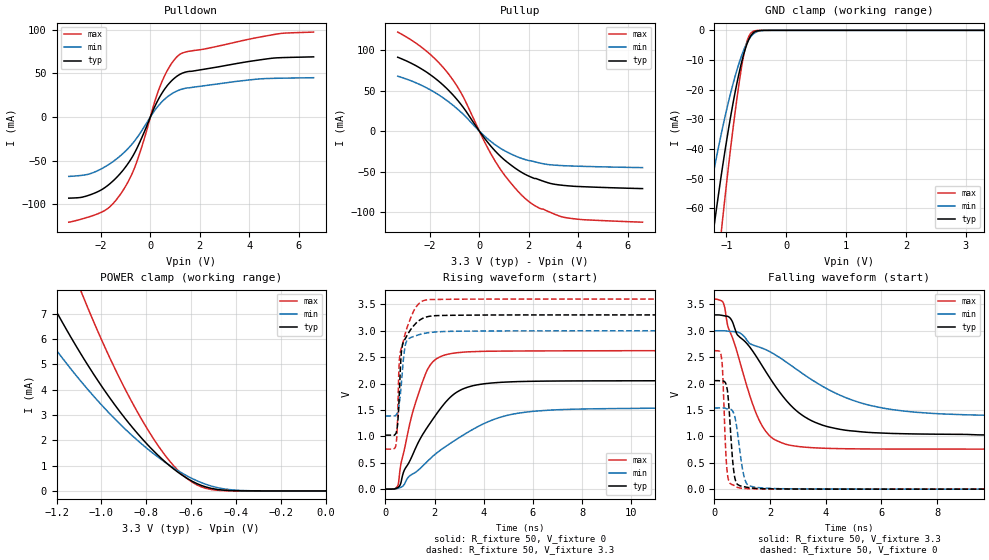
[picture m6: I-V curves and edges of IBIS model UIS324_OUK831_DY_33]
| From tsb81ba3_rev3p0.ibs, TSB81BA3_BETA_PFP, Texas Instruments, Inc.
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[Model]   UIS324_OUK831_DY_33
Model_type  I/O
Enable   Active-High
Vref =   0
Rref =   500
Cref =   10p
Vmeas =   1.65
| variable   typ   min   max
C_comp   1.99pF   1.39pF   3.76pF
| C_pullup   4.47pF   1.97pF   5.41pF
| C_pulldown   4.68pF   1.34pF   7.39pF
| C_tri-state   1.99pF   1.39pF   3.76pF
[Temperature Range]   40   125   -40
| Ambient temperature   25   110   -40
[Voltage range]   3.3   3   3.6
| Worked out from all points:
|   slope of the pulldown table from 0 to 0.495 V, typ, clamps not added: 17.4 ohm
|   slope of the pullup table from 0 to 0.495 V, typ, clamps not added: 25.3 ohm
|   GND clamp passes 1 mA (typ) near -0.56 V on its own axis
|   POWER clamp passes 1 mA (typ) near -0.70 V on its own axis
|   rising waveform, R_fixture 50, V_fixture 0: 20-80 % time 1.61ns typ, 2.77ns min, 911ps max; typ from 0 V to 2.05 V
|   falling waveform, R_fixture 50, V_fixture 3.3: 20-80 % time 1.97ns typ, 3.17ns min, 1.07ns max; typ from 3.3 V to 1.02 V
|   rising waveform, R_fixture 50, V_fixture 3.3: 20-80 % time 269ps typ, 202ps min, 369ps max; typ from 1.02 V to 3.3 V
|   falling waveform, R_fixture 50, V_fixture 0: 20-80 % time 172ps typ, 251ps min, 122ps max; typ from 2.06 V to 0 V
[GND Clamp]
| UIS324_OUK831_DY_33
|   Voltage   I(typ)   I(min)   I(max)
-3.3V     -469.1mA   -362mA     -576.5mA
-1.37V    -91.67mA   -65.2mA    -126.2mA
-1.2V     -65.15mA   -46.31mA   -90.59mA
-1.075V   -47.4mA    -33.88mA   -65.94mA
-890mV    -24.65mA   -18.1mA    -33.19mA
-755mV    -11.51mA   -9.042mA   -13.44mA
-710mV    -8.016mA   -6.622mA   -8.258mA
-660mV    -4.805mA   -4.37mA    -3.988mA
-615mV    -2.636mA   -2.778mA   -1.66mA
-560mV    -1.011mA   -1.412mA   -419uA
-370mV    -8.971uA   -44.43uA   -567.6nA
3.3V      178.8pA    2.977uA    41.06pA
[POWER Clamp]
| UIS324_OUK831_DY_33
|   Voltage   I(typ)   I(min)   I(max)
-3.3V     62.69mA    47.71mA    84.81mA
-1.38V    10.2mA     7.846mA    15.06mA
-1.235V   7.649mA    5.974mA    11.27mA
-1.095V   5.463mA    4.371mA    7.978mA
-1.075V   5.175mA    4.159mA    7.541mA
-940mV    3.397mA    2.844mA    4.835mA
-810mV    1.977mA    1.775mA    2.665mA
-705mV    1.063mA    1.064mA    1.279mA
-615mV    478.5uA    576.7uA    465.9uA
-535mV    157.4uA    262.1uA    102.8uA
-415mV    10.56uA    38.74uA    2.662uA
-48.03fV  178.8pA    6.248nA    49.98pA
[Pulldown]
| UIS324_OUK831_DY_33
|   Voltage   I(typ)   I(min)   I(max)
-3.3V     -92.9mA    -68.01mA   -120.4mA
-2.64V    -90.95mA   -66.29mA   -115.7mA
-1.855V   -81.13mA   -57.35mA   -107.2mA
-1.135V   -61.96mA   -42.51mA   -85.32mA
-570mV    -37.32mA   -24.91mA   -52.89mA
-240mV    -16.71mA   -10.9mA    -24.29mA
180mV     12mA       7.632mA    17.88mA
445mV     26.17mA    16.7mA     38.83mA
790mV     39.4mA     25.18mA    58.31mA
1.15V     48.05mA    30.64mA    70.82mA
5.11V     67.66mA    44.28mA    94.91mA
6.6V      68.79mA    44.92mA    97.14mA
[Pullup]
| UIS324_OUK831_DY_33
|   Voltage   I(typ)   I(min)   I(max)
-3.3V     91.06mA    67.68mA    122.1mA
-2.15V    73.02mA    53.59mA    98.88mA
-1.67V    62.17mA    45.17mA    85.36mA
-1.245V   50.31mA    36.14mA    70.38mA
-680mV    30.42mA    21.53mA    43.84mA
200mV     -8.419mA   -5.848mA   -12.61mA
710mV     -26.75mA   -18.34mA   -40.44mA
1.4V      -44.59mA   -29.91mA   -68.56mA
2V        -55.49mA   -36.31mA   -86.83mA
2.47V     -60.52mA   -39.5mA    -95.64mA
3.465V    -67.12mA   -42.73mA   -106.5mA
6.6V      -70.9mA    -45.03mA   -112.3mA
[Ramp]
| UIS324_OUK831_DY_33
| variable   typ   min   max
dV/dt_r   1.23/1.61E-09   0.92/2.77E-09   1.57/9.12E-10
dV/dt_f   1.37/1.97E-09   0.97/3.18E-09   1.71/1.08E-09
R_load = 50
[Rising Waveform]
| UIS324_OUK831_DY_33
R_fixture =   50
C_fixture =   0
L_fixture =   0
V_fixture =   0
V_fixture_min = 0
V_fixture_max = 0
|   Time   V(typ)   V(min)   V(max)
0s        -12.26uV   -75.17uV   -342.6nV
510ps     33.03mV    16.49mV    79.44mV
635ps     134.2mV    36.49mV    492.6mV
1.05ns    592.8mV    272.4mV    1.357V
1.71ns    1.177V     528.4mV    2.265V
2.11ns    1.446V     693.8mV    2.479V
2.81ns    1.808V     920.1mV    2.578V
4.72ns    2.024V     1.368V     2.615V
7.07ns    2.048V     1.505V     2.619V
40ns      2.054V     1.537V     2.623V
[Falling Waveform]
| UIS324_OUK831_DY_33
R_fixture =   50
C_fixture =   0
L_fixture =   0
V_fixture =   3.3
V_fixture_min = 3
V_fixture_max = 3.6
|   Time   V(typ)   V(min)   V(max)
0s        3.3V       3V         3.6V
330ps     3.285V     3V         3.512V
495ps     3.268V     2.991V     3.063V
1.695ns   2.353V     2.674V     1.218V
2.13ns    1.997V     2.562V     948mV
2.935ns   1.49V      2.275V     813.3mV
3.89ns    1.211V     1.946V     776.1mV
5.225ns   1.089V     1.639V     762.6mV
8.2ns     1.04V      1.424V     758.8mV
40ns      1.023V     1.384V     758.2mV
[Rising Waveform]
| UIS324_OUK831_DY_33
R_fixture =   50
C_fixture =   0
L_fixture =   0
V_fixture =   3.3
V_fixture_min = 3
V_fixture_max = 3.6
|   Time   V(typ)   V(min)   V(max)
0s        1.023V     1.384V     758.2mV
425ps     1.057V     1.4V       835.2mV
480ps     1.176V     1.444V     1.187V
555ps     1.722V     1.602V     2.359V
625ps     2.447V     1.887V     2.639V
755ps     2.809V     2.565V     2.858V
860ps     2.896V     2.802V     3.033V
1.23ns    3.137V     2.905V     3.439V
1.635ns   3.257V     2.955V     3.581V
40ns      3.3V       3V         3.6V
[Falling Waveform]
| UIS324_OUK831_DY_33
R_fixture =   50
C_fixture =   0
L_fixture =   0
V_fixture =   0
V_fixture_min = 0
V_fixture_max = 0
|   Time   V(typ)   V(min)   V(max)
0s        2.055V     1.538V     2.623V
190ps     2.052V     1.538V     2.609V
270ps     2.049V     1.538V     2.414V
415ps     1.989V     1.527V     627.4mV
490ps     1.751V     1.52V      207.4mV
705ps     304.1mV    1.421V     70.78mV
955ps     58.17mV    559.4mV    18.65mV
1.21ns    31.68mV    74.89mV    9.232mV
2.205ns   5.178mV    10.8mV     2.161mV
40ns      2.615uV    3.119uV    2.023uV
